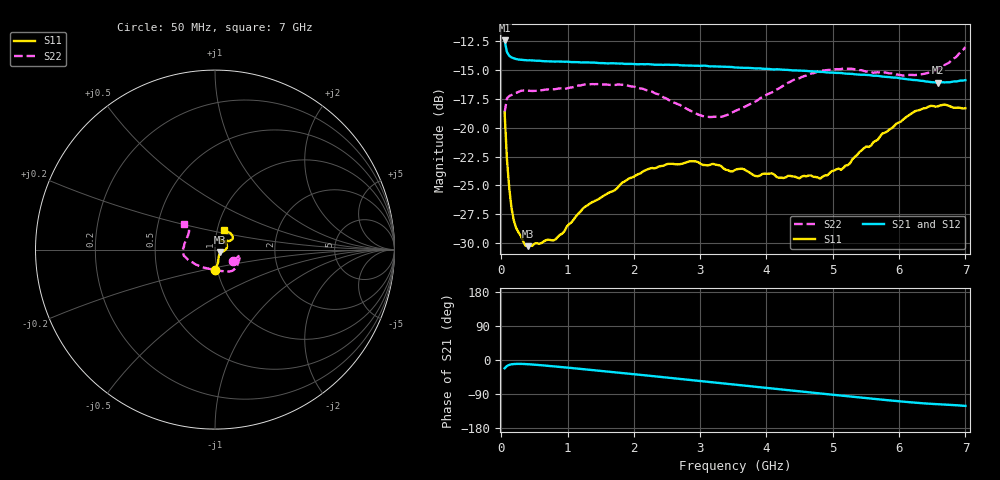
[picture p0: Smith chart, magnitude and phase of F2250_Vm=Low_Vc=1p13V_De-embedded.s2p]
! Integrated Device Technology
! Corporate Headquarters
! 6024 Silver Creek Valley Road
! San Jose, CA 95138  USA
! Phone:  1-408-284-8200
! Toll Free:  1-800-223-1366
! Webpage:  http://www.idt.com/
! Timing and RF Division
! 515 Groton Road, Suite 102
! Westford, MA 01886-6024
! Device:  F2250
! Description: Voltage Variable RF Attenuator
! Frequency:  50.0 -  6000.00 MHz
! Package:  3x3 mm Thin QFN Plastic Package: 16 pin
! Ports:  2 RF, 3 DC
!  Pin  1  = GND
!  Pin  2  = NC
!  Pin  3  = RF1  = Port 1
!  Pin  4  = NC
!  Pin  5  = GND
!  Pin  6  = GND
!  Pin  7  = GND
!  Pin  8  = GND
!  Pin  9  = NC
!  Pin 10  = RF2  = Port 2
!  Pin 11  = NC
!  Pin 12  = GND
!  Pin 13  = GND
!  Pin 14  = VCNTRL
!  Pin 15  = VDD
!  Pin 16  = VMODE
! Vcntrl:  1.130 Volts
! Vmode:  +0.000 Volts
! Vdd:  +3.30  Volts
! Current:  1.193 mA
! Data:  The device was measured on a the F2250 evaluation board which has
!  individual transmission lines to the RF pins.  Data was collected
!  using a calibrated network analyzer.  The evaluation board was
!  de-embedded using a TRL calibration technique.
!  The reference plane is the edge of the package pin.
! Misc:  SN 10
!  Action Tracker AT0258
! Date Measured:  2014-11-26
! Date:  2015-10-15  MJV
! Note:
!  Integrated Device Technology supplies this data as a sample of measured
!  data at the package pin for this product.  Your particular data for this
!  product may vary.
!  Data was taken at 25 degrees C.
!  Integrated Device Technology reserves the right to change this data at anytime.
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# GHz S dB R 50
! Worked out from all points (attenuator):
!   201 points, 50 MHz to 7 GHz, reference 50 ohm
!   highest |S21| = -12.43 dB at 50 MHz (marker M1); lowest = -16.1 dB at 6.583 GHz (marker M2)
!   lowest |S11| = -30.3 dB at 397.5 MHz (marker M3), VSWR 1.06, Z = 52.7 - j1.69 ohm
!   |S11| at or under -10 dB: start of sweep to end of sweep
!   |S22| runs from -19.1 to -13.0 dB; largest |S21 - S12| = 0.00078
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0.05  -18.69 -90.2  -12.43 -21.8  -12.43 -21.8  -18.68 -33.0
0.08475  -22.68 -76.6  -13.42 -15.8  -13.42 -15.8  -17.44 -17.5
0.1195  -25.22 -69.1  -13.76 -12.9  -13.75 -12.9  -17.25 -13.3
0.15425  -26.96 -62.7  -13.89 -11.4  -13.89 -11.4  -17.16 -12.1
0.22375  -28.69 -48.5  -14.04 -10.3  -14.05 -10.3  -16.97 -12.4
0.3975  -30.27 -31.5  -14.15 -11.1  -14.15 -11.1  -16.78 -14.5
0.8145  -29.70 -17.7  -14.26 -17.1  -14.24 -17.1  -16.65 -26.8
1.2315  -27.00 -13.9  -14.33 -24.1  -14.32 -24.1  -16.27 -37.5
1.857  -24.67 -0.9  -14.46 -34.9  -14.45 -34.9  -16.28 -50.0
2.37825  -23.35 11.7  -14.53 -44.1  -14.54 -44.1  -17.12 -61.7
2.86475  -22.90 27.0  -14.61 -52.9  -14.61 -52.9  -18.55 -80.9
3.0385  -23.22 33.2  -14.61 -56.1  -14.62 -56.1  -18.99 -90.6
3.3165  -23.33 43.6  -14.69 -61.2  -14.69 -61.2  -19.04 -108.5
3.525  -23.66 49.5  -14.77 -64.9  -14.77 -64.9  -18.55 -121.4
3.83775  -24.19 60.3  -14.86 -70.6  -14.83 -70.6  -17.71 -137.8
4.7065  -24.26 62.2  -15.10 -86.4  -15.10 -86.4  -15.27 -166.8
4.81075  -24.41 58.3  -15.16 -88.2  -15.15 -88.2  -15.05 -168.7
5.1235  -23.64 48.3  -15.25 -93.9  -15.26 -93.9  -14.91 -175.7
5.85325  -20.15 30.4  -15.61 -106.5  -15.61 -106.6  -15.28 167.4
6.2355  -18.58 32.4  -15.86 -112.5  -15.86 -112.6  -15.43 154.7
6.583  -18.15 41.5  -16.10 -116.6  -16.09 -116.7  -14.89 143.7
7  -18.30 65.0  -15.87 -121.1  -15.86 -121.2  -13.01 140.1
